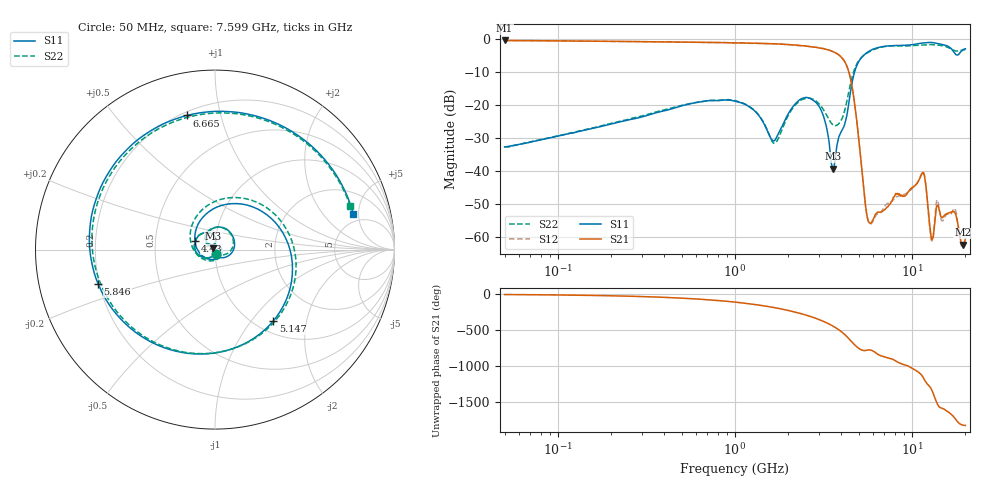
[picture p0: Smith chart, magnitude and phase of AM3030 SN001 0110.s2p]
# Hz S DB R 50
!freq MagS11 AngS11 MagS21 AngS21 MagS12 AngS12 MagS22 AngS22
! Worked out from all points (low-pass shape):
!   1601 points, 50 MHz to 20.05 GHz, reference 50 ohm
!   highest |S21| = -0.39 dB at 50 MHz (marker M1); lowest = -62.2 dB at 19.39 GHz (marker M2)
!   |S21| within 3 dB of the highest: start of sweep to 3.439 GHz
!   lowest |S11| = -39.2 dB at 3.605 GHz (marker M3), VSWR 1.02, Z = 49.1 + j0.66 ohm
!   |S11| at or under -10 dB: start of sweep to 4.738 GHz
!   |S22| runs from -32.6 to -1.6 dB; largest |S21 - S12| = 0.014
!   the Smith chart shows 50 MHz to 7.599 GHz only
!   S11 on the Smith chart (normalised r, x): 50 MHz: 1.01, -0.05; 4.43 GHz: 0.79, +0.08; 5.147 GHz: 1.20, -1.29; 5.846 GHz: 0.20, -0.14; 6.665 GHz: 0.22, +0.79; 7.599 GHz: 3.93, +4.30
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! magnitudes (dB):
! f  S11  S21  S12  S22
! 50 MHz  -32.6  -0.4  -0.4  -32.6
! 135.9 MHz  -27.8  -0.6  -0.6  -27.6
! 369.6 MHz  -22.1  -0.8  -0.8  -21.8
! 1.005 GHz  -18.8  -1.1  -1.1  -18.6
! 1.673 GHz  -30.7  -1.4  -1.4  -31.5
! 2.207 GHz  -19.4  -1.8  -1.9  -19.8
! 2.722 GHz  -18.2  -2.3  -2.3  -18.0
! 3.162 GHz  -23.2  -2.9  -2.8  -21.3
! 3.605 GHz  -39.2  -3.8  -3.8  -26.1
! 4.43 GHz  -18.3  -10.5  -10.5  -15.1
! 5.147 GHz  -5.8  -36.4  -36.5  -5.8
! 5.526 GHz  -4.2  -52.2  -52.2  -4.4
! 5.846 GHz  -3.4  -55.7  -56.0  -3.6
! 6.665 GHz  -2.3  -52.4  -52.4  -2.5
! 7.402 GHz  -2.0  -50.3  -49.7  -2.1
! 7.599 GHz  -2.0  -49.5  -49.3  -2.0
! 11.52 GHz  -1.2  -40.3  -40.0  -1.8
! 12.89 GHz  -1.0  -60.3  -60.9  -1.6
! 13.99 GHz  -1.3  -50.3  -48.9  -1.8
! 17.45 GHz  -4.3  -52.5  -51.3  -3.5
! 19.39 GHz  -3.2  -62.2  -62.2  -3.3
! 20.05 GHz  -2.9  -60.3  -60.8  -3.2
